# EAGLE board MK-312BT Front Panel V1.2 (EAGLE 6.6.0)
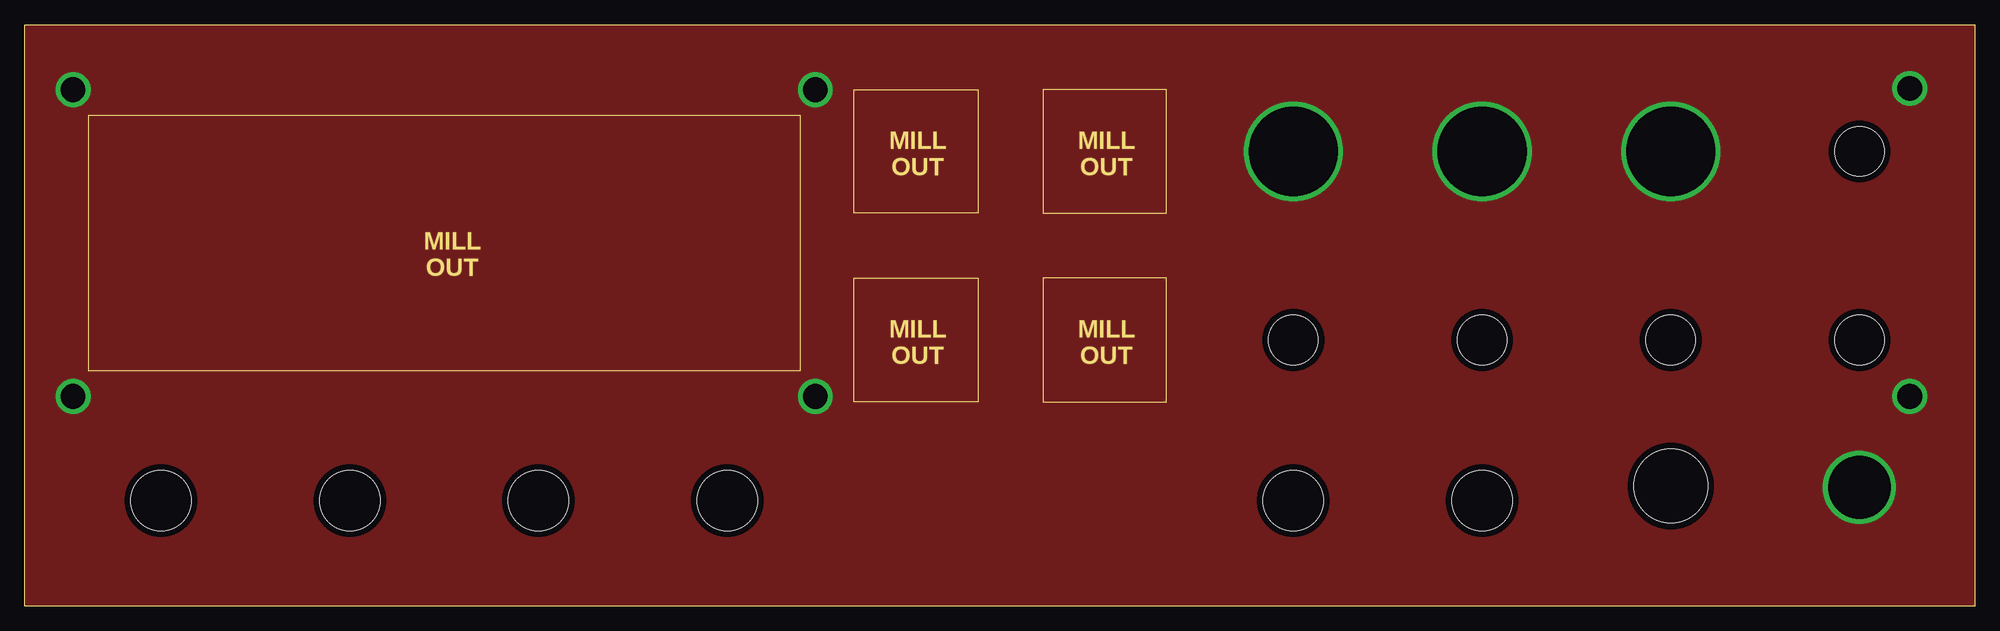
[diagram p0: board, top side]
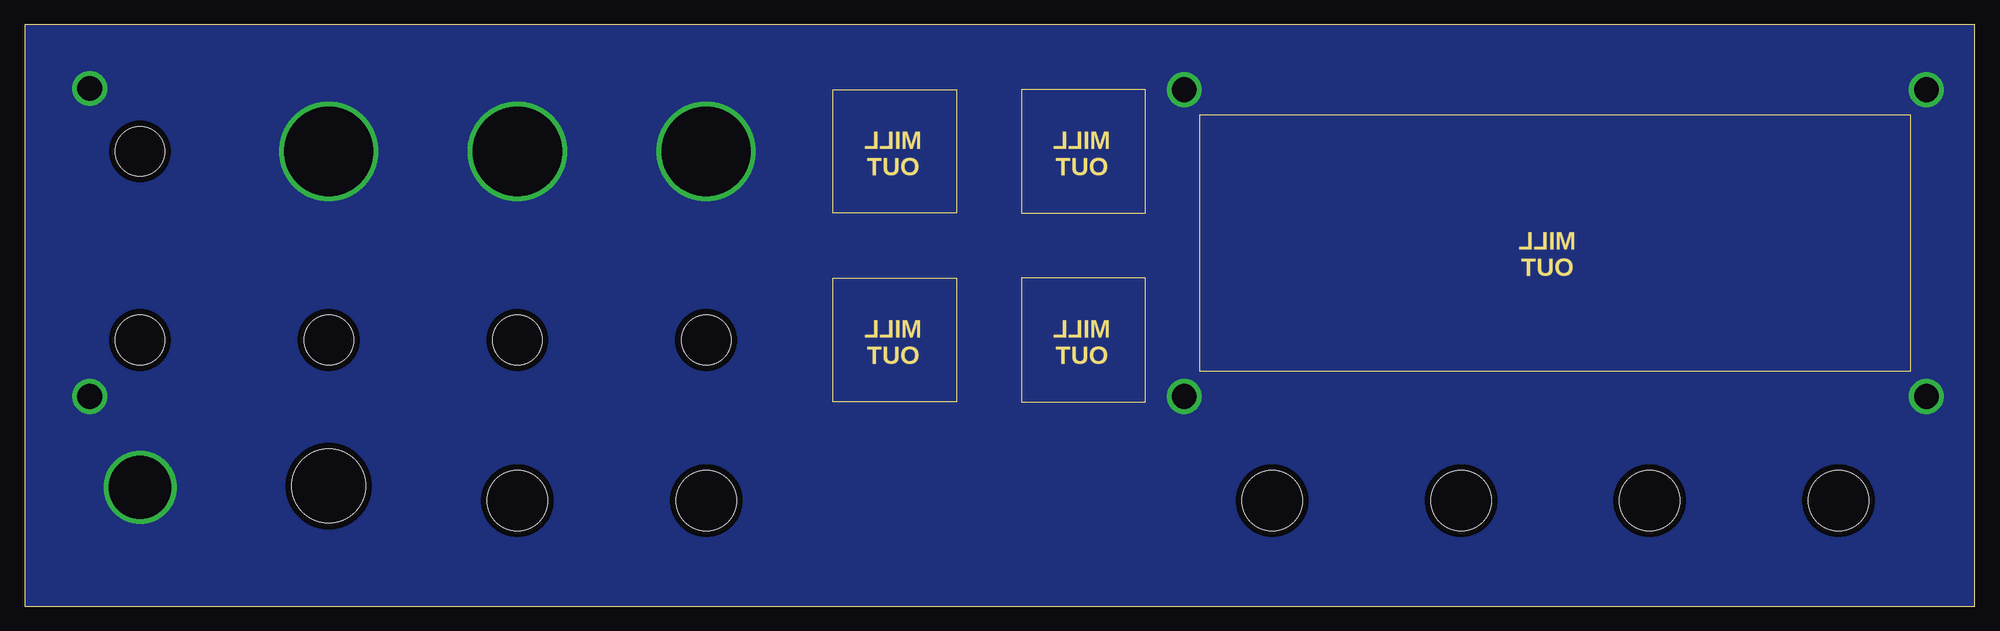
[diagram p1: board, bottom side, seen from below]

Size 196.85 x 58.72 mm. Coordinates in mm from the lower left corner, seen from the top.
Outline: 0,0 0,58.73 196.85,58.73 196.85,0 0,0
Copper layers (1*16): Top 0.035mm / dielectric 1.5mm / Bottom 0.035mm
Design rules "default *": minimum track width 10mil, minimum drill 24mil, track to track 8mil, track to pad 8mil, pad to pad 8mil, via to via 8mil, smd to smd 8mil, copper to edge 0mil, drill to drill 10mil, minimum pad ring 10mil, minimum via ring 8mil, stop-mask expansion 4mil, vias tented up to drill 0mil, thermal gap 10mil
Holes 5 mm at 128.07,26.89 147.12,26.89 185.22,26.89 166.17,26.89 185.22,45.94
Holes 6.1 mm at 13.77,10.64 32.82,10.64 51.87,10.64 70.92,10.64 128.07,10.64 147.12,10.64
Holes 7.5 mm at 166.17,12.14
Milling: 20 lines

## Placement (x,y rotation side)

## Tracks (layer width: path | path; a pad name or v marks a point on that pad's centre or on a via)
GND  (via drill 2.5, 6.35, 9)
  other vias: 4.88,21.17 4.88,52.17 79.81,52.17 79.81,21.17 128.07,45.94 147.12,45.94 166.17,45.94 185.22,11.99 190.3,21.17 190.3,52.29
  pour Top (isolate 0.61): 0,0 0,58.72 196.85,58.72 196.85,0
  pour Bottom (isolate 0.61): 0,0 0,58.72 196.85,58.72 196.85,0

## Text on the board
tStop: MENU | LEVEL | MULTI | LCD | A | B | ADJUST | ACTIVITY | RADIO | POWER | A | B | OK | - | + | ON | INPUTS | OUTPUTS | MK-312BT | MIC | LINE | REMOTE | LINK | A | B | VDC | OFF
Milling: MILL / OUT | MILL / OUT | MILL / OUT | MILL / OUT | MILL / OUT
